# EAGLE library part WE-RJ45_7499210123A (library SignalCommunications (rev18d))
Order Code 7499210123A Design THT xBase-T 10/100 Base-T PoE Ports 1x1 Application PoE Tab Position VERTICAL LED (Left-Right) YELLOW-GREEN EMI Fingers No Details see: http://katalog.we-online.de/en/pbs/WE-LAN_RJ45/7499210123? Updated by Yingchun Shan 2016-08-30 2016(C) Würth Elektronik
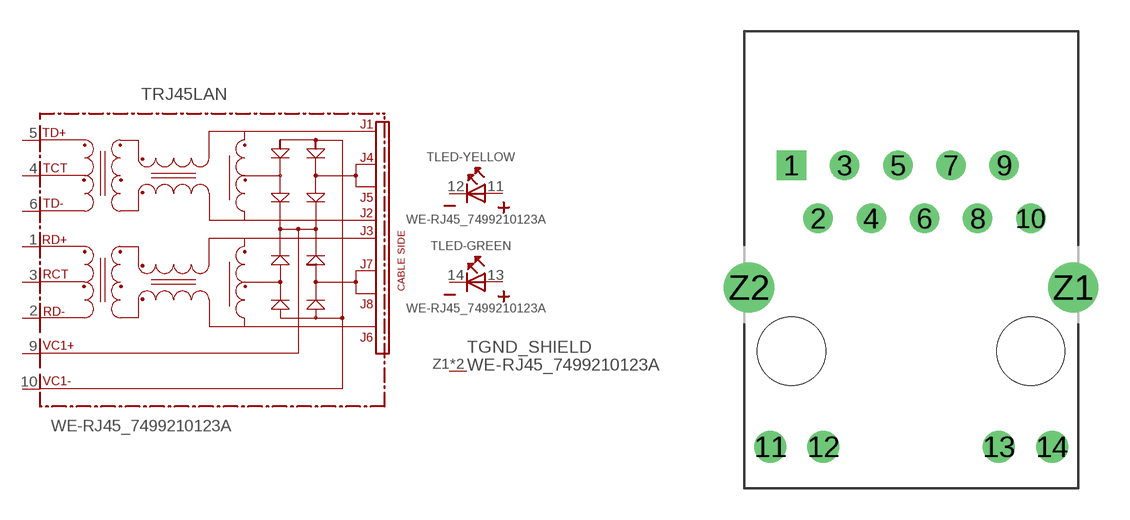
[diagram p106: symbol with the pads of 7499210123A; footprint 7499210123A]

Designator prefix T; gates LED-YELLOW=LED2PIN LED-GREEN=LED2PIN RJ45LAN=749921-THT-POE-RVS GND_SHIELD=GND_PIN

## WE-RJ45_7499210123A (COMPANY-URL: http://www.we-online.de; CREATED-BY: Christin Zierenner; CREATED-DATE: AUG 2012; DATASHEET-URL: http://katalog.we-online.de/kataloge/eisos/media/pdf/7499210123.pdf; MANUFACTURER: Würth Elektronik eiSos GmbH)  [7499210123A]
1  RJ45LAN:RD+
2  RJ45LAN:RD-
3  RJ45LAN:RCT
4  RJ45LAN:TCT
5  RJ45LAN:TD+
6  RJ45LAN:TD-
9  RJ45LAN:VC1+  pwr
10  RJ45LAN:VC1-  pwr
11  LED-YELLOW:A  pas
12  LED-YELLOW:K  pas
13  LED-GREEN:A  pas
14  LED-GREEN:K  pas
Z1  GND_SHIELD:1  pwr
Z2  GND_SHIELD:1  pwr

## Footprint 7499210123A (pad centres in mm)
MAX HEIGHT=16.90mm PORTS----1X1 LED ---YES
drill 0.9 square: 1 -5.715,8.89
drill 0.9: 2 -4.445,6.35; 3 -3.175,8.89; 4 -1.905,6.35; 5 -0.635,8.89; 6 0.635,6.35; 7 1.905,8.89; 8 3.175,6.35; 9 4.445,8.89; 10 5.715,6.35
drill 1.02: 11 -6.73,-4.57; 12 -4.19,-4.57; 13 4.19,-4.57; 14 6.73,-4.57
drill 1.6: Z1 7.745,3.05; Z2 -7.745,3.05
hole 3.25 at -5.715,0
hole 3.25 at 5.715,0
